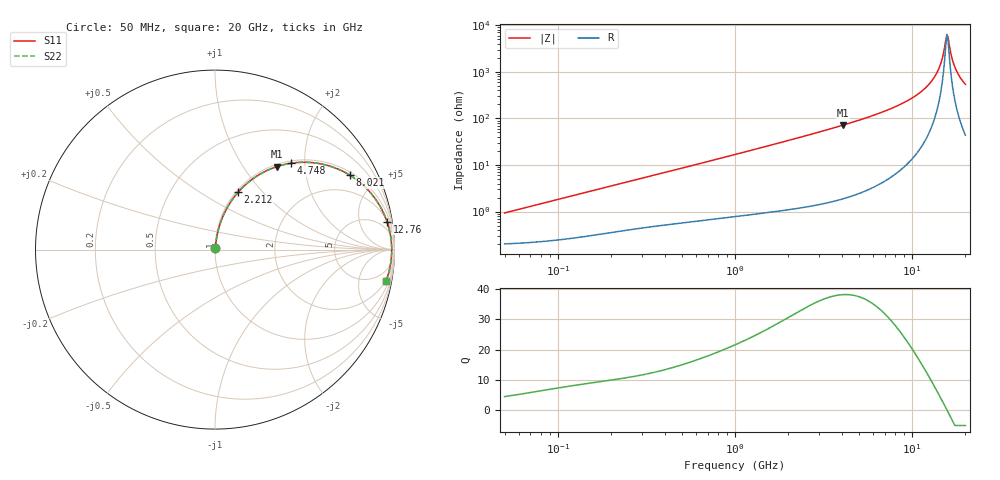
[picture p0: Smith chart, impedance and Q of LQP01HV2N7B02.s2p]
!Murata Part Number: LQP01HV2N7B02
!These Parameters are Measured in Series Mode Connection
!  o--[Z]--o
!Port1  Port2
!  o-------o
!Freq. Start=50[MHz] Stop=20[GHz], 401[Steps]
# Hz S RI R 50
!Freq.(Hz) S11(Real) S11(Imag) S21(Real) S21(Imag) S12(Real) S12(Imag) S22(Real) S22(Imag)
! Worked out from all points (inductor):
!   401 points, 50 MHz to 20 GHz, reference 50 ohm
!   read as one part in series: L = 2.9 nH near 51.52 MHz
!   highest Q = 38.2 at 4.088 GHz (marker M1), where L = 2.8 nH
!   self-resonance near 15.74 GHz
!   S11 on the Smith chart (normalised r, x): 50 MHz: 1.00, +0.02; 2.212 GHz: 1.02, +0.74; 4.748 GHz: 1.05, +1.71; 8.021 GHz: 1.13, +3.54; 12.76 GHz: 2, +12; 20 GHz: 2, -11
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5e7  0.0021 0.00909  0.9979 -0.00909  0.9979 -0.00909  0.0021 0.00909
1.364002e8  0.00343 0.0243  0.9966 -0.0243  0.9966 -0.0243  0.00343 0.0243
3.721004e8  0.00894 0.063  0.9911 -0.063  0.9911 -0.063  0.00894 0.063
1e9  0.0343 0.1604  0.9657 -0.1604  0.9657 -0.1604  0.0343 0.1604
2.211938e9  0.1289 0.3199  0.8711 -0.3199  0.8711 -0.3199  0.1289 0.3199
2.728004e9  0.1829 0.3726  0.8171 -0.3726  0.8171 -0.3726  0.1829 0.3726
4.087748e9  0.3442 0.4622  0.6558 -0.4622  0.6558 -0.4622  0.3442 0.4622
4.748272e9  0.4245 0.4812  0.5755 -0.4812  0.5755 -0.4812  0.4245 0.4812
7.442007e9  0.7043 0.4401  0.2957 -0.4401  0.2957 -0.4401  0.7043 0.4401
8.020766e9  0.7503 0.4154  0.2497 -0.4154  0.2497 -0.4154  0.7503 0.4154
1.050288e10  0.8922 0.284  0.1078 -0.284  0.1078 -0.284  0.8922 0.284
1.276073e10  0.9583 0.1561  0.0417 -0.1561  0.0417 -0.1561  0.9583 0.1561
1.417136e10  0.9776 0.0801  0.0224 -0.0801  0.0224 -0.0801  0.9776 0.0801
1.482269e10  0.9821 0.0467  0.0179 -0.0467  0.0179 -0.0467  0.9821 0.0467
1.550395e10  0.9843 0.013  0.0157 -0.013  0.0157 -0.013  0.9843 0.013
1.573793e10  0.9845 0.00176  0.0155 -0.00176  0.0155 -0.00176  0.9845 0.00176
1.597544e10  0.9845 -0.00949  0.0155 0.00949  0.0155 0.00949  0.9845 -0.00949
1.621653e10  0.9842 -0.0207  0.0158 0.0207  0.0158 0.0207  0.9842 -0.0207
1.696185e10  0.9817 -0.0544  0.0183 0.0544  0.0183 0.0544  0.9817 -0.0544
1.774144e10  0.9769 -0.0878  0.0231 0.0878  0.0231 0.0878  0.9769 -0.0878
1.88369e10  0.967 -0.1316  0.033 0.1316  0.033 0.1316  0.967 -0.1316
2e10  0.9532 -0.1743  0.0468 0.1743  0.0468 0.1743  0.9532 -0.1743
